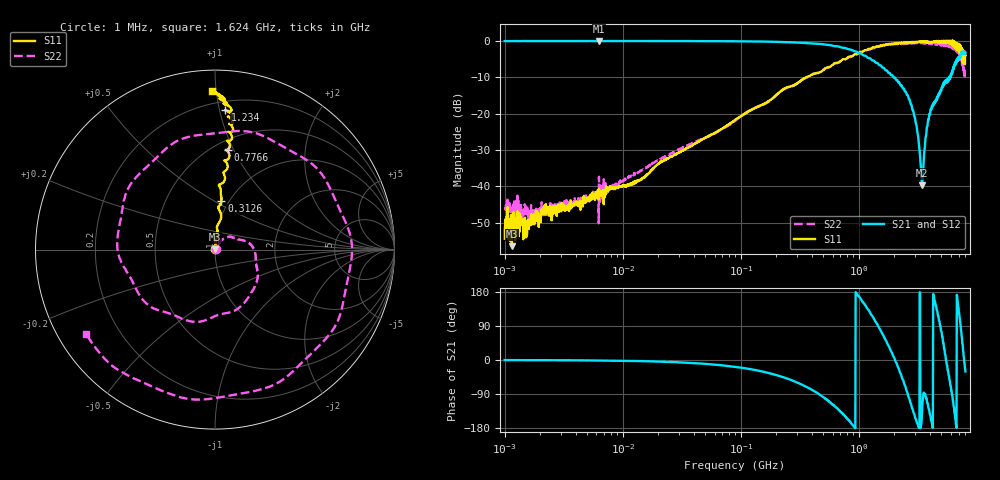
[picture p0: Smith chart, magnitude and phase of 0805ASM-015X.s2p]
!s-Parameter Generated by FASTRON Sdn. Bhd.
!FASTRON P/N : 0805ASM-015X
!Keysight Technologies: E5071C_MY46733604_B.14.02
!Date: Fri Jun 19 14:47:45 2026
!Version  :Rev00  Fri Jun 19 14:47:45 2026
!Data & Calibration Information:
!Freq  S11:SOLT2(ON)  S21:SOLT2(ON)  S12:SOLT2(ON)  S22:SOLT2(ON)
!PortZ  Port1:50+j0  Port2:50+j0
!When reading reference impedance value at option line is always used.
! Remarks : This data is being provided solely for informational purposes.
# Hz S dB R 50
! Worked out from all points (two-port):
!   1601 points, 1 MHz to 8 GHz, reference 50 ohm
!   highest |S21| = 0.00 dB at 6.301 MHz (marker M1); lowest = -39.7 dB at 3.426 GHz (marker M2)
!   |S21| within 3 dB of the highest: start of sweep to 961.8 MHz; 7.600198 GHz to 7.63 GHz (29.8 MHz wide, 0.391 % of centre)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
!   lowest |S11| = -56.5 dB at 1.152 MHz (marker M3), VSWR 1.00, Z = 50.1 + j0.0711 ohm
!   |S11| at or under -10 dB: start of sweep to 360.1 MHz
!   |S22| runs from -50.2 to -0.4 dB; largest |S21 - S12| = 0.014
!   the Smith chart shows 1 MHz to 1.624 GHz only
!   S11 on the Smith chart (normalised r, x): 1 MHz: 1.00, +0.00; 312.6 MHz: 0.92, +0.54; 776.6 MHz: 0.58, +0.95; 1.234 GHz: 0.26, +1.04; 1.624 GHz: 0.12, +0.98
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1000000  -54.40 19.3  -0.06 -0.3  -0.03 -0.2  -46.60 12.3
1151819  -56.50 28.3  -0.06 -0.3  -0.03 -0.2  -45.80 14.8
4479405  -44.90 50.1  -0.05 -0.9  -0.04 -1.0  -44.30 50.0
6301378  -40.70 53.9  -0.00 -1.5  -0.02 -1.3  -37.40 49.4
2.00676e7  -33.80 79.1  -0.06 -4.1  -0.06 -4.0  -32.80 65.7
8.994653e7  -21.70 81.0  -0.11 -18.1  -0.11 -18.1  -21.90 51.2
3.126022e8  -11.30 82.5  -0.48 -61.8  -0.48 -61.8  -11.20 -29.7
4.006501e8  -9.32 84.9  -0.71 -78.6  -0.71 -78.6  -9.23 -64.1
7.765934e8  -5.01 82.7  -2.02 -151.0  -2.02 -151.0  -4.98 156.0
1.233539e9  -2.17 85.9  -4.73 128.0  -4.74 128.0  -2.41 -11.9
1.624461e9  -1.06 91.0  -7.40 63.2  -7.43 63.0  -1.32 -147.0
1.7949e9  -0.86 95.3  -8.83 37.0  -8.82 36.8  -0.99 155.0
2.199693e9  -0.51 109.0  -11.50 -26.2  -11.50 -26.4  -0.88 14.8
2.516241e9  -0.42 116.0  -14.20 -77.4  -14.20 -77.5  -0.84 -96.9
3.029771e9  -0.45 124.0  -22.40 -155.0  -22.40 -155.0  -0.47 89.9
3.42643e9  -0.36 145.0  -39.70 -144.0  -39.70 -144.0  -0.43 -43.7
3.791269e9  -0.28 151.0  -23.60 -112.0  -23.60 -112.0  -0.68 -173.0
4.075033e9  -0.29 153.0  -18.70 -155.0  -18.70 -156.0  -0.82 88.2
4.57657e9  -0.24 172.0  -15.90 131.0  -16.00 130.0  -0.73 -82.7
5.136407e9  -0.07 -150.0  -12.10 57.9  -12.20 57.4  -1.28 88.6
5.668252e9  -0.62 -150.0  -11.10 -27.5  -11.10 -27.4  -1.13 -77.4
8e9  -3.85 -61.9  -3.19 -30.1  -3.02 -30.0  -9.05 -135.0
